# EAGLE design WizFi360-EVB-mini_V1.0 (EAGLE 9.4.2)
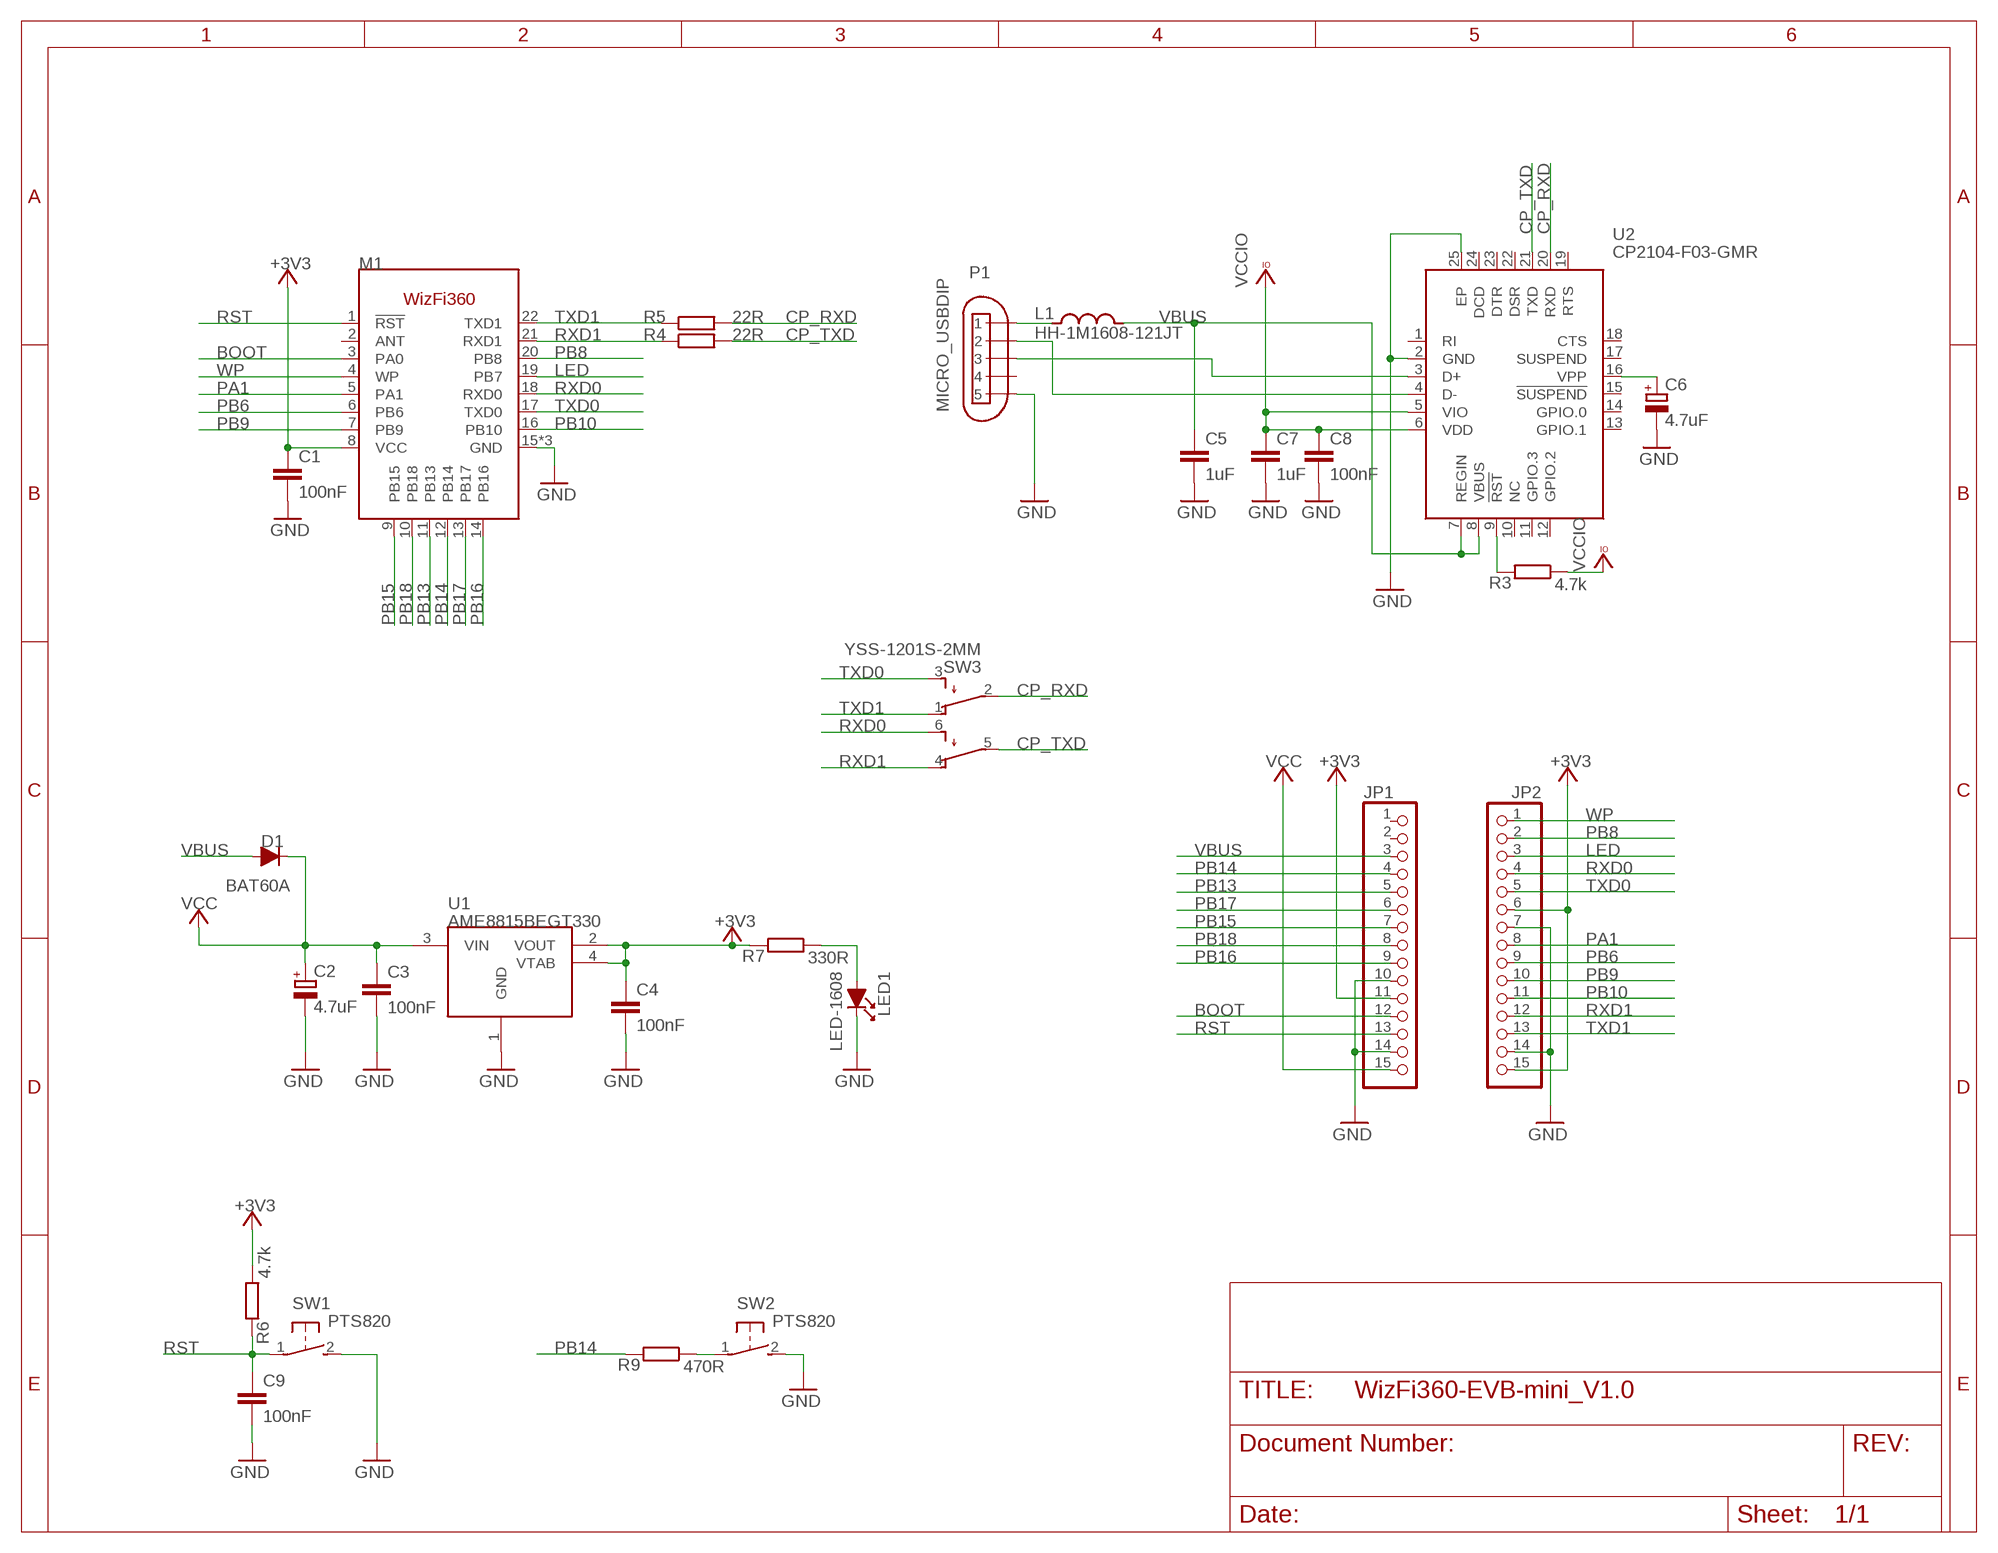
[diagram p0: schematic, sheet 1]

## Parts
C1  100nF  0142_10NF_0603  [C0603-ROUND@1]
C2  4.7uF  0474_TAJA475M016RNJ  [SMC_A]
C3  100nF  0142_10NF_0603  [C0603-ROUND@1]
C4  100nF  0142_10NF_0603  [C0603-ROUND@1]
C5  1uF  0142_10NF_0603  [C0603-ROUND@1]
C6  4.7uF  0474_TAJA475M016RNJ  [SMC_A]
C7  1uF  0142_10NF_0603  [C0603-ROUND@1]
C8  100nF  0142_10NF_0603  [C0603-ROUND@1]
C9  100nF  0142_10NF_0603  [C0603-ROUND@1]
D1  BAT60A  [BAT60A]
JP1  PINHD-1X15  [1X15]
JP2  PINHD-1X15  [1X15]
L1  HH-1M1608-121JT  BLM18PG471SN1D  [0603-1608X90N]
LED1  LED-1608  [LED-1608]
M1  WIZFI360  [WIZFI360]
P1  MICRO_USBDIP  [MICRO_USB_D]
R3  4.7k  0028_CR0603JW103L  [R0603-ROUND]
R4  22R  0028_CR0603JW103L  [R0603-ROUND]
R5  22R  0028_CR0603JW103L  [R0603-ROUND]
R6  4.7k  0028_CR0603JW103L  [R0603-ROUND]
R7  330R  0028_CR0603JW103L  [R0603-ROUND]
R9  470R  0028_CR0603JW103L  [R0603-ROUND]
SW1  PTS820  [PTS820]
SW2  PTS820  [PTS820]
SW3  YSS-1201S-2MM  [YSS-1201S-2MM]
U1  AME8815BEGT330  [SOT-223]
U2  CP2104-F03-GMR  [QFN50P400X400X80-25N]

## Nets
+3V3 [power]: C1.1 C4.1 JP1.11 JP2.6 JP2.15 M1.8(VCC) R6.1 R7.2 U1.2(VOUT) U1.4(VTAB)
BOOT: JP1.12 M1.3(PA0)
CP_RXD: R5.2 SW3.2(P) U2.20(RXD)
CP_TXD: R4.2 SW3.5(P1) U2.21(TXD)
GND: C1.2 C2.- C3.2 C4.2 C5.2 C6.- C7.2 C8.2 C9.2 JP1.10 JP1.14 JP2.7 JP2.14 LED1.K M1.15(GND) M1.23(GND) M1.24(GND) P1.5 P1.GND1 P1.GND2 P1.GND3 P1.GND4 P1.GND5 P1.GND6 SW1.2(S) SW2.2(S) U1.1(GND) U2.2(GND) U2.25(EP)
LED: JP2.3 M1.19(PB7)
N$1: L1.1 P1.1
N$4: P1.3 U2.3(D+)
N$5: P1.2 U2.4(D-)
N$6: C6.+ U2.16(VPP)
N$7: LED1.A R7.1
N$8: R3.2 U2.9(!RST)
N$9: R9.1 SW2.1(P)
PA1: JP2.8 M1.5(PA1)
PB6: JP2.9 M1.6(PB6)
PB8: JP2.2 M1.20(PB8)
PB9: JP2.10 M1.7(PB9)
PB10: JP2.11 M1.16(PB10)
PB13: JP1.5 M1.11(PB13)
PB14: JP1.4 M1.12(PB14) R9.2
PB15: JP1.7 M1.9(PB15)
PB16: JP1.9 M1.14(PB16)
PB17: JP1.6 M1.13(PB17)
PB18: JP1.8 M1.10(PB18)
RST: C9.1 JP1.13 M1.1(!RST!) R6.2 SW1.1(P)
RXD0: JP2.4 M1.18(RXD0) SW3.6(S1)
RXD1: JP2.12 M1.21(RXD1) R4.1 SW3.4(O1)
TXD0: JP2.5 M1.17(TXD0) SW3.3(S)
TXD1: JP2.13 M1.22(TXD1) R5.1 SW3.1(O)
VBUS: C5.1 D1.2 JP1.3 L1.2 U2.7(REGIN) U2.8(VBUS)
VCC: C2.+ C3.1 D1.1 JP1.15 U1.3(VIN)
VCCIO: C7.1 C8.1 R3.1 U2.5(VIO) U2.6(VDD)
WP: JP2.1 M1.4(WP)
Unconnected: JP1.1 JP1.2 M1.2(ANT) P1.4 U2.1(RI) U2.10(NC) U2.11(GPIO.3) U2.12(GPIO.2) U2.13(GPIO.1) U2.14(GPIO.0) U2.15(!SUSPEND) U2.17(SUSPEND) U2.18(CTS) U2.19(RTS) U2.22(DSR) U2.23(DTR) U2.24(DCD)

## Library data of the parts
C1 C3-C5 C7-C9 = Condensatori:0142_10NF_0603: 10nF 0603; CASE: 0603; MONTHLY_USAGE: _____; PART_NUMBER: 10nF_0603; PRICE: _____; SUPPLIER: _____; TYPE: Condensatori; VALUE: 10nF
C2 C6 = Condensatori:0474_TAJA475M016RNJ: 4u7 tantalio Case A - testa gialla -Tantalio; CASE: CaseA_(1206); MONTHLY_USAGE: _____; PART_NUMBER: TAJA475M016RNJ; PRICE: _____; SUPPLIER: _____; TYPE: Condensatori; VALUE: 4u7
D1 = DIODE:BAT60A
JP1 JP2 = PinHeader:PINHD-1X15: PIN HEADER
L1 = MK1_Zero:BLM18PG471SN1D: FERRITE CHIP 470 OHM 1000MA 0603
LED1 = DIODE:LED-1608
M1 = WIZnet:WIZFI360
P1 = Connector:MICRO_USB
R3-R7 R9 = Resistenze:0028_CR0603JW103L: 10K 0603; CASE: 0603; MONTHLY_USAGE: _____; PART_NUMBER: CR0603JW103L; PRICE: _____; SUPPLIER: _____; TYPE: Resistenze; VALUE: 10k
SW1 SW2 = Switch:PTS820
SW3 = Switch:YSS-1201S-2MM
U1 = RECULATOR:AME8815BEGT330
U2 = untitled:CP2104-F03-GMR: USB-to-UART 1-CH 576byte FIFO 3.3V Automotive 24-Pin QFN EP T/R Source: Datasheet; DESCRIPTION: USB-to-UART 1-CH 576byte FIFO 3.3V Automotive 24-Pin QFN EP T/R; HEIGHT: 0.8mm; MANUFACTURER_NAME: Silicon Labs; MANUFACTURER_PART_NUMBER: CP2104-F03-GMR; MOUSER_PART_NUMBER: 634-CP2104-F03-GMR; MOUSER_PRICE-STOCK: https://www.mouser.com/Search/Refine.aspx?Keyword=634-CP2104-F03-GMR

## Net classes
0 default: width 0.203 mm, drill 0.008 mm, clearance 0.127 mm
1 power: width 0.305 mm, drill 0.3 mm, clearance 0.203 mm

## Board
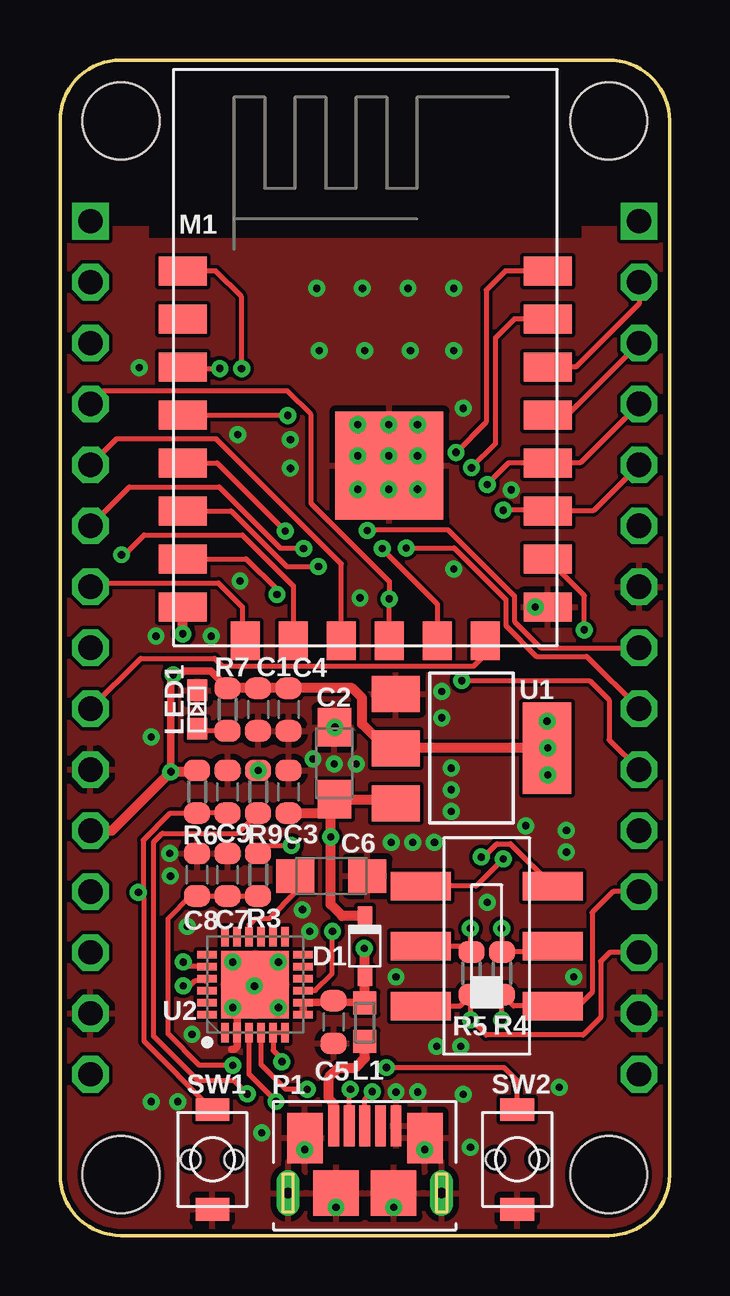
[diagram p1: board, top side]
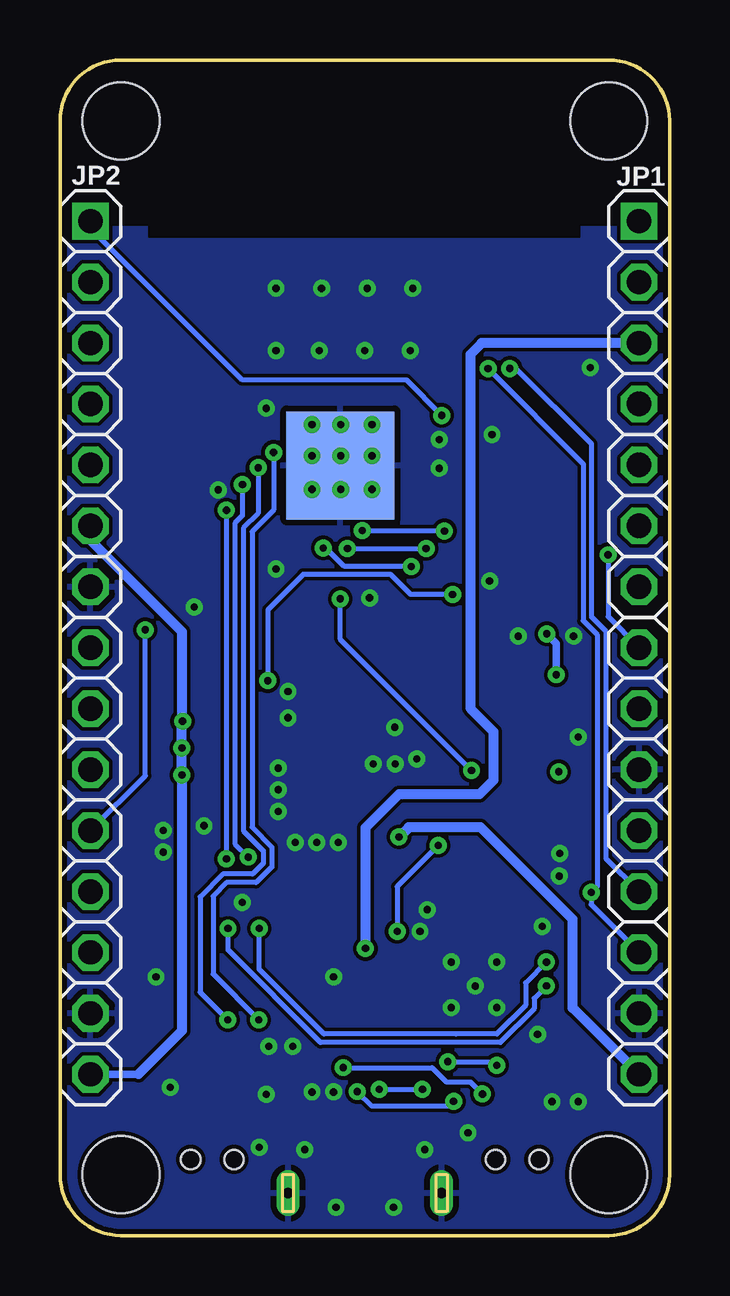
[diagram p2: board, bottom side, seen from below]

Size 25.4 x 49 mm. Coordinates in mm from the lower left corner, seen from the top.
Outline: 0,2.54 0,46.46 arc-90 2.54,49 22.86,49 arc-90 25.4,46.46 25.4,2.54 arc-90 22.86,0 2.54,0 arc-90 0,2.54
Copper layers (1*16): Top 0.035mm / dielectric 1.5mm / Bottom 0.035mm
Design rules "default *": minimum track width 6mil, minimum drill 0.35mm, track to track 6mil, track to pad 6mil, pad to pad 5mil, via to via 6mil, smd to smd 6mil, copper to edge 8mil, drill to drill 1mil, minimum pad ring 10mil, minimum via ring 8mil, stop-mask expansion 6mil, vias tented up to drill 15mil, thermal gap 10mil
Holes 3.2 mm at 2.54,2.54 22.86,2.54 22.86,46.46 2.54,46.46

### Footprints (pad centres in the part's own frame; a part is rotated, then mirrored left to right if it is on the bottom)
C0603-ROUND@1 = smd 0.898 x 1.1: 1 -0.889,0; 2 0.889,0
SMC_A = smd 1.6 x 1.4: + -1.5,0; - 1.5,0
BAT60A = smd 0.8 x 0.6: 1 1.25,0; 2 -1.25,0
1X15 = drill 1.016 square: 1 -17.78,0 | drill 1.016 octagon: 2 -15.24,0; 3 -12.7,0; 4 -10.16,0; 5 -7.62,0; 6 -5.08,0; 7 -2.54,0; 8 0,0; 9 2.54,0; 10 5.08,0; 11 7.62,0; 12 10.16,0; 13 12.7,0; 14 15.24,0; 15 17.78,0
0603-1608X90N = smd 0.95 x 1: 1 -0.8,0; 2 0.8,0
LED-1608 = smd 0.89 x 0.82: A -0.8,0; K 0.8,0
WIZFI360 = smd 2 x 1.2: 1 -7.6,3.6; 2 -7.6,1.6; 3 -7.6,-0.4; 4 -7.6,-2.4; 5 -7.6,-4.4; 6 -7.6,-6.4; 7 -7.6,-8.4; 8 -7.6,-10.4; 15 7.6,-10.4; 16 7.6,-8.4; 17 7.6,-6.4; 18 7.6,-4.4; 19 7.6,-2.4; 20 7.6,-0.4; 21 7.6,1.6; 22 7.6,3.6 | smd 1.2 x 1.6: 9 -5,-11.8; 10 -3,-11.8; 11 -1,-11.8; 12 1,-11.8; 13 3,-11.8; 14 5,-11.8 | smd 4.5 x 4.5: 23 1,-4.5 | smd 4.5 x 4.5 bottom: 24 1,-4.5
MICRO_USB_D = smd 1.7 x 0.45: 1 2.8,1.3; 2 2.8,0.65; 3 2.8,0; 4 2.8,-0.65; 5 2.8,-1.3 | drill 0.45 long: GND1 0,3.2; GND4 0,-3.2 | smd 2.1 x 1.475: GND2 2.3,2.5; GND3 2.3,-2.5 | smd 1.9 x 1.9: GND5 0,-1.2; GND6 0,1.2
R0603-ROUND = smd 0.898 x 1.1: 1 -0.889,0; 2 0.889,0
PTS820 = smd 0.95 x 1.4: 1 -2.075,0; 2 2.075,0 | hole 0.8: 0,0.9; 0,-0.9
YSS-1201S-2MM = smd 1.2 x 2.5: 1 -2.5,2.75; 2 0,2.75; 3 2.5,2.75; 4 -2.5,-2.75; 5 0,-2.75; 6 2.5,-2.75
SOT-223 = smd 1.499 x 2.007: 1 -2.261,-3.15; 2 0.025,-3.15; 3 2.311,-3.15 | smd 3.81 x 2.007: 4 0,3.15
QFN50P400X400X80-25N = smd 0.8 x 0.3: 1 -2,1.25; 2 -2,0.75; 3 -2,0.25; 4 -2,-0.25; 5 -2,-0.75; 6 -2,-1.25; 13 2,-1.25; 14 2,-0.75; 15 2,-0.25; 16 2,0.25; 17 2,0.75; 18 2,1.25 | smd 0.3 x 0.8: 7 -1.25,-2; 8 -0.75,-2; 9 -0.25,-2; 10 0.25,-2; 11 0.75,-2; 12 1.25,-2; 19 1.25,2; 20 0.75,2; 21 0.25,2; 22 -0.25,2; 23 -0.75,2; 24 -1.25,2 | smd 2.8 x 2.8: 25 0,0

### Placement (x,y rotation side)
C1  8.26,21.93 270 top
C2  11.43,19.68 90 top
C3  9.53,18.5 90 top
C4  9.53,21.93 270 top
C5  11.4,8.9 270 top
C6  11.3,14.99 0 top
C7  6.99,15.04 90 top
C8  5.71,15.04 90 top
C9  6.99,18.5 90 top
D1  12.7,12.06 90 top
JP1  1.27,24.5 270 bottom
JP2  24.13,24.5 270 bottom
L1  12.7,8.89 90 top
LED1  5.71,21.93 90 top
M1  12.72,36.6 0 top
P1  12.7,1.77 90 top
R3  8.26,15.04 90 top
R4  18.41,10.93 90 top
R5  17.14,10.93 90 top
R6  5.71,18.5 270 top
R7  6.99,21.93 90 top
R9  8.26,18.5 90 top
SW1  6.35,3.17 270 top
SW2  19.05,3.17 270 top
SW3  17.78,12.06 90 top
U1  17.14,20.32 270 top
U2  8.13,10.46 90 top
U$1  [WIZFI_LOGO]  20,42.4 0 bottom

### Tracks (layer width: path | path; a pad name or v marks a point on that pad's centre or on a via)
+3V3  (via drill 0.3)
  Top 0.305: v4.62,19.33 4.62,23.27 v4.72,23.38 5.01,23.38 5.16,23.53 6.27,23.53 R7.2 | U1.4 v20.32,20.32
  Top 0.406: U1.4 13.48,20.32 13.4,20.4 13.89,20.4 U1.2 13.61,20.3 12.59,21.31 12.59,22.4 12.17,22.81 C4.1 C1.1 R7.2 | v5.12,25.08 M1.8 | JP1.11 2.17,16.88 v4.62,19.33 5.66,19.33 R6.1
  Bottom 0.305: v5.12,25.08 4.72,24.68 v4.72,23.38 | 22.13,6.72 JP2.15
  Bottom 0.406: JP2.6 24.13,28.98 20.32,25.17 20.32,21.46 v20.3,21.44 20.32,21.41 v20.32,20.32 v20.32,19.2 20.32,8.53 22.13,6.72
BOOT  (via drill 0.3)
  Top 0.203: 5.12,36.6 M1.3 5.12,36.14 v6.66,36.14
  Bottom 0.203: v6.66,36.14 6.4,36.14 3.25,32.99 3.25,25.78 2.64,25.17 2.64,15.7 2.63,15.7 JP1.12
CP_RXD  (via drill 0.3)
  Top 0.203: U2.20 5.32,11.21 v5.13,11.4 | SW3.2 16.9,12.06 17.03,11.93 | 17.03,11.93 R5.2 | v17.1,12.8 17.1,12 17.03,11.93
  Bottom 0.203: v5.13,11.4 6,10.53 6,9.6 7.2,8.4 8.89,8.4 14.4,8.4 17.1,11.1 v17.1,12.8
CP_TXD  (via drill 0.3)
  Top 0.203: U2.21 6.03,10.61 5.62,10.61 5.41,10.4 v5.13,10.4 | SW3.5 20.28,11.82 R4.2 18.4,11.83 v18.4,12.8
  Bottom 0.203: v5.13,10.4 5.64,9.89 5.64,9.45 7.05,8.04 14.55,8.04 18.4,11.9 v18.4,12.8
GND  (via drill 0.3)
  Top 0.305: v7.2,9.5 7.38,9.32 U2.2 7.38,7.88 7.26,7.76 7.16,7.76 | M1.24 14.9,33.68 v14.9,33.8 | v13.7,31.1 13.72,31.12 M1.24 | M1.24 13.72,32.28 v14.9,31.1 | M1.24 v12.4,32.5 | M1.24 v13.7,32.5 v12.4,33.8 | M1.24 13.72,32.42 v12.4,31.1
  other vias: 8.1,10.4 9.1,11.4 7.2,11.4 9.1,9.5 14.9,32.5 13.7,33.8 11.43,19.66 15.9,22.68 4.57,15.93 11.46,21.18 12.34,19.66 10.54,19.86 9.6,33.18 7.4,33.38 9.6,31.98 12.5,26.58 16.4,27.78 18.8,31.08 14.7,16.38 16.3,18.58 19.4,17.08 20.8,6.18 16.8,5.88 11.5,1.18 13.9,1.18 15.2,3.58 10.2,3.58 6.3,24.98 12.7,36.88 14.6,36.88 10.8,36.88 10.7,39.48 12.6,39.48 14.5,39.48 15.9,21.58 3.8,20.78 4.9,5.58 3.8,5.58 8.4,4.28 17.1,3.68 21.4,10.78 14,10.78 21.1,15.98 10.1,13.58 5.3,12.88 5.5,8.38 16.7,7.88 15.7,7.88 3.3,36.18 7.5,27.28 21.1,16.88 16.3,17.68 15.6,16.38 13.8,16.38 10.4,12.68 14,5.98 14.9,5.98 19.8,26.2 4.6,14.98 16.3,19.48 16.4,39.48 16.4,36.88 4,24.98 17.8,13.88 16.8,34.48
  pour Top: 0,0 0,42 26,42 26,0
  pour Bottom: -1,-1 27,-1 27,42 -1,42
LED
  Top 0.203: JP2.3 21.13,34.2 M1.19
N$1
  Top 0.406: P1.1 11.4,5.5 11.2,5.7 11.2,6.59 11.61,7 12.3,7 12.7,7.4 L1.1
N$4  (via drill 0.3)
  Top 0.203: P1.3 12.7,5.69 v13.01,6 | v9,5.59 7.88,6.71 U2.3
  Bottom 0.203: v13.01,6 12.41,5.4 9.19,5.4 v9,5.59
N$5  (via drill 0.3)
  Top 0.203: P1.2 12.05,6.05 v12.1,6.1 | v10.3,6.1 9.4,6.1 8.38,7.12 U2.4
  Bottom 0.203: v12.1,6.1 v10.3,6.1
N$6
  Top 0.203: C6.+ 9.8,14.3 8.71,13.21 8.13,13.21 7.88,12.96 U2.16
N$7
  Top 0.203: R7.1 5.8,21.04 LED1.A
N$8  (via drill 0.3)
  Top 0.203: U2.9 10.64,10.21 11.32,10.9 11.32,12.64 v11.35,12.68 | R3.2 8.58,16.26 v9.64,16.26
  Bottom 0.203: v9.64,16.26 11.35,14.55 v11.35,12.68
N$9  (via drill 0.3)
  Top 0.203: SW2.1 19.05,6.45 18.5,7 v13.6,7 | R9.1 7.41,16.76 4.26,16.76 3.9,16.4 3.9,8.3 5.75,6.45 7.25,6.45 v7.8,5.9
  Bottom 0.203: v7.8,5.9 8.3,6.4 9.3,6.4 9.9,7 v13.6,7
PA1  (via drill 0.3)
  Top 0.203: M1.5 6.55,32.2 v9.38,29.37 | v12.8,29.39 12.83,29.41 16.18,29.41 18.93,26.66 18.93,25.6 20.03,24.5 JP2.8
  Bottom 0.203: v9.38,29.37 12.78,29.37 v12.8,29.39
PB6  (via drill 0.3)
  Top 0.203: M1.6 7.13,30.2 9.45,27.88 v10.76,27.88 v10.77,27.88 | v14.43,28.66 16.42,28.66 18.57,26.51 18.57,25.42 19.85,24.14 21.95,24.14 JP2.9
  Bottom 0.203: v14.43,28.66 14.33,28.66 13.58,27.91 10.79,27.91 v10.77,27.88
PB8
  Top 0.203: JP2.2 24.13,38.84 21.49,36.2 M1.20
PB9  (via drill 0.3)
  Top 0.203: M1.7 7.76,28.2 9.04,26.92 v9.04,26.72 | v16.74,23.13 22.07,23.13 22.89,22.31 22.89,20.66 JP2.10
  Bottom 0.203: v9.04,26.72 10.79,26.72 11.63,27.55 15.27,27.55 16.74,26.08 v16.74,23.13
PB10  (via drill 0.3)
  Top 0.203: v21.84,25.25 21.84,26.67 M1.16
  Bottom 0.203: JP2.11 21.84,19.17 v21.84,25.25
PB13
  Top 0.203: M1.11 11.72,28 6.52,33.2 2.35,33.2 JP1.5
PB14  (via drill 0.3)
  Top 0.203: JP1.4 1.81,35.2 9.47,35.2 10.46,34.21 10.46,30.52 13.72,27.26 v13.72,26.54 M1.12
  Bottom 0.203: v8.26,19.39 13.72,24.85 v13.72,26.54
PB15
  Top 0.203: JP1.7 1.43,27.2 6.6,27.2 7.6,26.2 7.6,25.32 M1.9
PB16
  Top 0.203: M1.14 17.72,24.22 17.23,23.73 6.77,23.73 6.44,24.06 3.37,24.06 JP1.9
PB17  (via drill 0.3)
  Top 0.203: JP1.6 2.89,31.2 6.63,31.2 9.19,28.64 v10.15,28.64 | M1.13 15.72,26.32 13.42,28.61 v13.42,28.64
  Bottom 0.203: v13.42,28.64 v10.15,28.64
PB18  (via drill 0.3)
  Top 0.203: v2.56,28.38 2.67,28.38 3.5,29.2 7.6,29.2 9.72,27.08 M1.10
  Bottom 0.203: JP1.8 2.56,25.79 v2.56,28.38
RST  (via drill 0.3)
  Top 0.203: 3.4,14.17 3.4,14.2 3.26,14.34 | SW1.1 3.5,8.1 3.5,14.07 3.4,14.17 | 3.4,14.17 v3.27,14.3 3.47,14.5 3.47,16.47 4.6,17.61 R6.2 C9.1 | v7.56,36.13 7.56,39.13 6.49,40.2 M1.1
  Bottom 0.203: v7.56,36.13 3.61,32.18 3.61,25.63 3,25.02 3,14.57 v3.27,14.3 3.27,13.8 JP1.13
RXD0  (via drill 0.3)
  Top 0.203: JP2.4 21.67,32.2 M1.18 18.68,32.2 17.8,31.32 v17.8,31.3 | v17.56,15.77 17.65,15.77 18.2,16.33 18.77,16.33 SW3.6
  Bottom 0.203: v17.8,31.3 17.8,30 18.11,29.69 18.11,16.33 v17.56,15.77
RXD1  (via drill 0.3)
  Top 0.203: M1.21 18.92,38.2 18.14,37.41 18.14,32.99 v17.14,32 | v18.41,8.99 R4.1 18.89,9.56 SW3.4 21.61,9.56 22.17,10.13 22.17,13.46 23.05,14.34 JP2.12
  Bottom 0.203: v17.14,32 17.14,30.1 17.75,29.49 17.75,16.86 16.93,16.04 16.93,15.51 17.37,15.06 18.61,15.06 19.56,14.12 19.56,10.14 v18.41,8.99
TXD0  (via drill 0.3)
  Top 0.203: JP2.5 22.21,30.2 M1.17 20.31,30.19 20.3,30.17 20.28,30.23 v18.47,30.23 | v18.47,15.7 17.33,14.56 SW3.3
  Bottom 0.203: v18.47,30.23 v18.47,15.7
TXD1  (via drill 0.3)
  Top 0.203: SW3.1 16.67,9.56 R5.1 17.12,10.02 v17.12,8.99 17.76,8.36 21.79,8.36 22.53,9.09 22.53,11.43 22.9,11.8 JP2.13 | M1.22 18.54,40.2 17.75,39.41 17.75,33.9 v16.5,32.65
  Bottom 0.203: v16.5,32.65 16.5,30.24 17.4,29.34 17.4,17.01 16.57,16.18 16.57,15.36 17.22,14.71 18.47,14.71 19.02,14.15 19.02,10.9 v17.12,8.99
VBUS  (via drill 0.3)
  Top 0.305: 11.32,9.71 U2.8 U2.7 | 11.32,9.71 C5.1 | L1.2 12.68,9.71 11.32,9.71
  Top 0.406: L1.2 D1.2 12.7,11.94 v12.68,11.96
  Bottom 0.406: v12.68,11.96 12.68,16.99 11.28,18.39 7.92,18.39 7.34,18.97 7.34,21.01 8.31,21.97 8.31,36.73 7.83,37.2 JP1.3
VCC  (via drill 0.3)
  Top 0.406: 12.62,13.39 D1.1 11.76,13.31 11.28,13.79 v11.28,16.61 11.28,18.03 C2.+ | 9.5,17.58 C3.1 10.85,17.61 C2.+ | C2.+ 13.82,18.18 U1.3
  Bottom 0.406: JP1.15 4.04,9.49 4.04,13.18 7.87,17.02 10.87,17.02 v11.28,16.61
VCCIO  (via drill 0.3)
  Top 0.203: v9.25,7.25 9.25,7.36 8.88,7.72 U2.5 U2.6 | v7.2,7.1 5.8,7.1 4.5,8.4 4.5,13.2 5.45,14.15 C8.1 C7.1 R3.1 7.99,14.15
  Bottom 0.203: v9.25,7.25 7.35,7.25 v7.2,7.1
WP  (via drill 0.3)
  Top 0.203: M1.4 5.13,34.19 v9.49,34.19
  Bottom 0.203: v9.49,34.19 10.96,35.66 17.8,35.66 24.13,41.99 JP2.1

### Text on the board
silk_top: WP | RSV | RSV | PB8 | RSV | LED | VBUS | RXD0 | PB14 | TXD0 | PB13 | 3V3 | PB17 | GND | PB15 | PA1 | PB18 | PB6 | PB16 | PB9 | GND | UART0 | PB10 | 3V3 | RXD1 | PA0 | TXD1 | RST | GND | UART1 | GND | 3V3 | Vin | RST | SW
silkbottom: RSV | WP | WizFi360-EVB-mini | RSV | PB8 | VBUS | LED | PB14 | RXD0 | PB13 | TXD0 | PB17 | 3V3 | PB15 | GND | PB18 | PA1 | PB16 | PB6 | GND | PB9 | 3V3 | PB10 | PA0 | RXD1 | RST | TXD1 | GND | GND | Vin | 3V3 | Version 1.0 | Made in KOREA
